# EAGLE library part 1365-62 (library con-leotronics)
DUAL ROW STRAIGHT HEADER 1364 SERIES. 1.27mm x 1.27mm. Without Fixing Post. SMT Source: http://www.leotronics.co.uk/Conexcon/Data%20Sheets/sec.%20A/1364ing.pdf
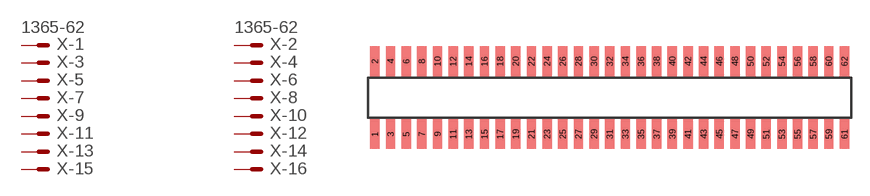
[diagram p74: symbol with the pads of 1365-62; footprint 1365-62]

Designator prefix X; gates -1=MVAL -2=MVAL -3=M -4=M -5=M -6=M -7=M -8=M -9=M -10=M -11=M -12=M -13=M -14=M -15=M -16=M -17=M -18=M -19=M -20=M -21=M -22=M -23=M -24=M -25=M -26=M -27=M -28=M -29=M -30=M -31=M -32=M -33=M -34=M -35=M -36=M -37=M -38=M -39=M -40=M -41=M -42=M -43=M -44=M -45=M -46=M -47=M -48=M -49=M -50=M -51=M -52=M -53=M -54=M -55=M -56=M -57=M -58=M -59=M -60=M -61=M -62=M

## 1365-62 (OC_FARNELL: unknown; OC_NEWARK: unknown)  [1365-62]
1  -1:S  pas
2  -2:S  pas
3  -3:S  pas
4  -4:S  pas
5  -5:S  pas
6  -6:S  pas
7  -7:S  pas
8  -8:S  pas
9  -9:S  pas
10  -10:S  pas
11  -11:S  pas
12  -12:S  pas
13  -13:S  pas
14  -14:S  pas
15  -15:S  pas
16  -16:S  pas
17  -17:S  pas
18  -18:S  pas
19  -19:S  pas
20  -20:S  pas
21  -21:S  pas
22  -22:S  pas
23  -23:S  pas
24  -24:S  pas
25  -25:S  pas
26  -26:S  pas
27  -27:S  pas
28  -28:S  pas
29  -29:S  pas
30  -30:S  pas
31  -31:S  pas
32  -32:S  pas
33  -33:S  pas
34  -34:S  pas
35  -35:S  pas
36  -36:S  pas
37  -37:S  pas
38  -38:S  pas
39  -39:S  pas
40  -40:S  pas
41  -41:S  pas
42  -42:S  pas
43  -43:S  pas
44  -44:S  pas
45  -45:S  pas
46  -46:S  pas
47  -47:S  pas
48  -48:S  pas
49  -49:S  pas
50  -50:S  pas
51  -51:S  pas
52  -52:S  pas
53  -53:S  pas
54  -54:S  pas
55  -55:S  pas
56  -56:S  pas
57  -57:S  pas
58  -58:S  pas
59  -59:S  pas
60  -60:S  pas
61  -61:S  pas
62  -62:S  pas

## Footprint 1365-62 (pad centres in mm)
DUAL ROW STRAIGHT HEADER 1364 SERIES. 1.27mm x 1.27mm. Without Fixing Post. SMT Source: http://www.leotronics.co.uk/Conexcon/Data%20Sheets/sec.%20A/1364ing.pdf
smd 0.76 x 2.4: 1 -19.05,-2.95; 2 -19.05,2.95; 3 -17.78,-2.95; 4 -17.78,2.95; 5 -16.51,-2.95; 6 -16.51,2.95; 7 -15.24,-2.95; 8 -15.24,2.95; 9 -13.97,-2.95; 10 -13.97,2.95; 11 -12.7,-2.95; 12 -12.7,2.95; 13 -11.43,-2.95; 14 -11.43,2.95; 15 -10.16,-2.95; 16 -10.16,2.95; 17 -8.89,-2.95; 18 -8.89,2.95; 19 -7.62,-2.95; 20 -7.62,2.95; 21 -6.35,-2.95; 22 -6.35,2.95; 23 -5.08,-2.95; 24 -5.08,2.95; 25 -3.81,-2.95; 26 -3.81,2.95; 27 -2.54,-2.95; 28 -2.54,2.95; 29 -1.27,-2.95; 30 -1.27,2.95; 31 0,-2.95; 32 0,2.95; 33 1.27,-2.95; 34 1.27,2.95; 35 2.54,-2.95; 36 2.54,2.95; 37 3.81,-2.95; 38 3.81,2.95; 39 5.08,-2.95; 40 5.08,2.95; 41 6.35,-2.95; 42 6.35,2.95; 43 7.62,-2.95; 44 7.62,2.95; 45 8.89,-2.95; 46 8.89,2.95; 47 10.16,-2.95; 48 10.16,2.95; 49 11.43,-2.95; 50 11.43,2.95; 51 12.7,-2.95; 52 12.7,2.95; 53 13.97,-2.95; 54 13.97,2.95; 55 15.24,-2.95; 56 15.24,2.95; 57 16.51,-2.95; 58 16.51,2.95; 59 17.78,-2.95; 60 17.78,2.95; 61 19.05,-2.95; 62 19.05,2.95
